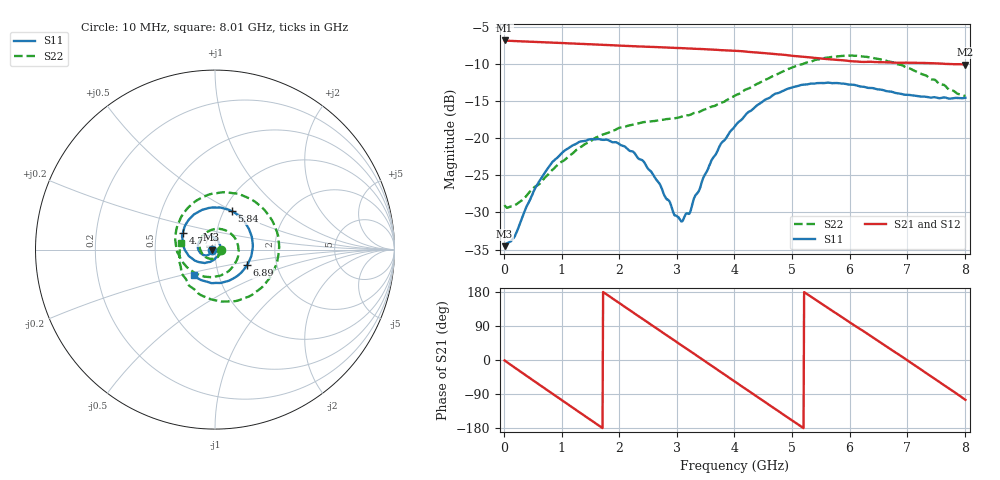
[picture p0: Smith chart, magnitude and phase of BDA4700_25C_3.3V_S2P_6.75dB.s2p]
!Agilent Technologies,E5071B,MY42404982,A.09.10
!Date: Mon Oct 20 18:05:50 2025
!Data & Calibration Information:
!Freq	S11:SOLT2(ON)	S21:SOLT2(ON)	S12:SOLT2(ON)	S22:SOLT2(ON)
# Hz S RI R 50
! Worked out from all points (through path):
!   801 points, 10 MHz to 8.01 GHz, reference 50 ohm
!   highest |S21| = -6.86 dB at 10 MHz (marker M1); lowest = -10.1 dB at 8.01 GHz (marker M2)
!   group delay of S21, straight-line fit = 285 ps
!   lowest |S11| = -34.5 dB at 10 MHz (marker M3), VSWR 1.04, Z = 48.2 - j0.0898 ohm
!   |S11| at or under -10 dB: start of sweep to end of sweep
!   |S22| runs from -29.4 to -8.9 dB; largest |S21 - S12| = 0.0052
!   S11 on the Smith chart (normalised r, x): 10 MHz: 0.96, -0.00; 4.77 GHz: 0.69, +0.13; 5.84 GHz: 1.09, +0.49; 6.89 GHz: 1.41, -0.25; 8.01 GHz: 0.76, -0.22
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1e7  -0.0187 -0.000932  0.4537 -0.00993  0.4536 -0.0102  0.0354 -0.00269
1.7e8  -0.0192 -0.00939  0.4267 -0.142  0.4268 -0.1417  0.0316 -0.0156
3.3e8  -0.0237 -0.0188  0.3649 -0.2584  0.3645 -0.2585  0.0239 -0.0304
7.2e8  -0.0499 -0.0324  0.1038 -0.4285  0.1038 -0.4283  -0.0179 -0.0517
1.02e9  -0.0772 -0.0227  -0.1326 -0.4149  -0.1328 -0.4152  -0.0603 -0.0355
1.35e9  -0.095 0.00747  -0.3399 -0.2637  -0.3399 -0.264  -0.0855 0.0207
1.64e9  -0.0896 0.0412  -0.4216 -0.0567  -0.4216 -0.0567  -0.0658 0.0784
1.93e9  -0.0656 0.0671  -0.3884 0.1606  -0.3886 0.1606  -0.00574 0.1134
2.32e9  -0.0195 0.0712  -0.1898 0.3679  -0.1899 0.3681  0.0888 0.0887
2.68e9  0.0176 0.0472  0.07 0.403  0.0692 0.4028  0.1318 -0.00139
3.1e9  0.0265 -0.00816  0.3229 0.2405  0.321 0.2423  0.0838 -0.1127
3.54e9  -0.0132 -0.0605  0.3911 -0.0585  0.3908 -0.059  -0.0452 -0.152
4.01e9  -0.101 -0.0657  0.2098 -0.3247  0.2102 -0.3241  -0.1795 -0.0714
4.38e9  -0.1645 -0.00828  -0.0356 -0.3749  -0.0356 -0.3759  -0.2216 0.0631
4.77e9  -0.1786 0.0933  -0.2623 -0.2547  -0.2609 -0.2559  -0.1626 0.2185
5.35e9  -0.0649 0.2234  -0.3356 0.0912  -0.3361 0.0893  0.096 0.3148
5.84e9  0.0952 0.213  -0.1444 0.3019  -0.1432 0.3016  0.3117 0.1729
6.25e9  0.1889 0.1153  0.0837 0.3148  0.0886 0.3133  0.35 -0.0494
6.68e9  0.2046 -0.0238  0.2748 0.1692  0.2754 0.1684  0.2246 -0.2387
6.89e9  0.1793 -0.0854  0.3155 0.0591  0.3158 0.0571  0.1245 -0.2849
7.52e9  0.0188 -0.1856  0.1865 -0.2577  0.1862 -0.2581  -0.1523 -0.1841
8.01e9  -0.1198 -0.1433  -0.0811 -0.302  -0.0803 -0.3024  -0.1882 0.0388
